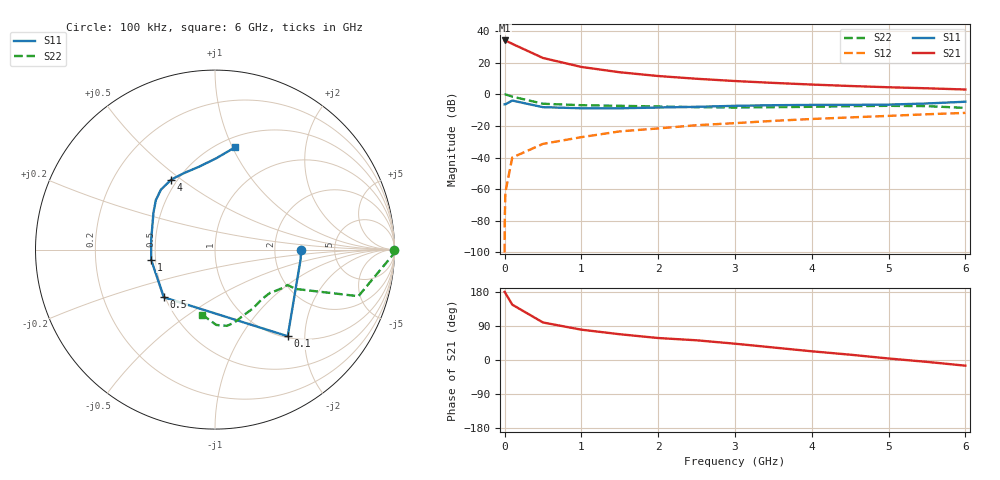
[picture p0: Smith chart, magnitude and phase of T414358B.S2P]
!AT-41435
!S-PARAMETERS at Vce=8V  Ic=25mA.  LAST UPDATED 07-21-92
# ghz s ma r 50
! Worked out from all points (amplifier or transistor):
!   16 points, 100 kHz to 6 GHz, reference 50 ohm
!   highest |S21| = 34.0 dB at 100 kHz (marker M1)
!   |S21| within 3 dB of that: start of sweep to 138.5 MHz
!   unconditionally stable (mu >= 1): start of sweep to 174.9 kHz; 797.4 MHz to 3.869 GHz
!   at 10 MHz: K = 0.18, MSG = 48.0 dB, |S12| = -61.9 dB
!   at 2.5 GHz: K = 1.11, MAG = 12.7 dB, |S12| = -19.6 dB
!   at 6 GHz: K = 0.81, MSG = 7.4 dB, |S12| = -11.8 dB
!   S11 on the Smith chart (normalised r, x): 100 kHz: 2.85, -0.01; 100 MHz: 1.03, -1.64; 500 MHz: 0.49, -0.31; 1 GHz: 0.47, -0.06; 4 GHz: 0.46, +0.46; 6 GHz: 0.60, +1.02
0.0001  0.48 -0.1  50 179.9  1e-05 85.0  0.999 0.0
0.001  0.48 -0.7  50 179.6  8e-05 89.0  0.999 -0.2
0.01  0.48 -6.8  50 176.6  0.0008 88.0  0.99 -1.8
0.1  0.63 -50.0  39.08 146.0  0.01 83.0  0.84 -18.0
0.5  0.39 -137.0  13.97 99.0  0.027 60.0  0.5 -26.0
1  0.36 -171.0  7.28 80.0  0.044 67.0  0.45 -26.0
1.5  0.36 171.0  4.94 68.0  0.067 66.0  0.43 -30.0
2  0.38 156.0  3.76 58.0  0.083 63.0  0.41 -34.0
2.5  0.4 149.0  3.08 52.0  0.105 63.0  0.39 -38.0
3  0.43 140.0  2.61 43.0  0.122 64.0  0.38 -47.0
3.5  0.45 132.0  2.28 33.0  0.144 59.0  0.39 -57.0
4  0.46 122.0  2.02 23.0  0.165 55.0  0.4 -67.0
4.5  0.46 112.0  1.82 14.0  0.185 50.0  0.42 -75.0
5  0.47 101.0  1.66 4.0  0.207 45.0  0.43 -81.0
5.5  0.51 89.0  1.54 -5.0  0.233 39.0  0.42 -89.0
6  0.58 79.0  1.41 -15.0  0.257 33.0  0.37 -101.0
